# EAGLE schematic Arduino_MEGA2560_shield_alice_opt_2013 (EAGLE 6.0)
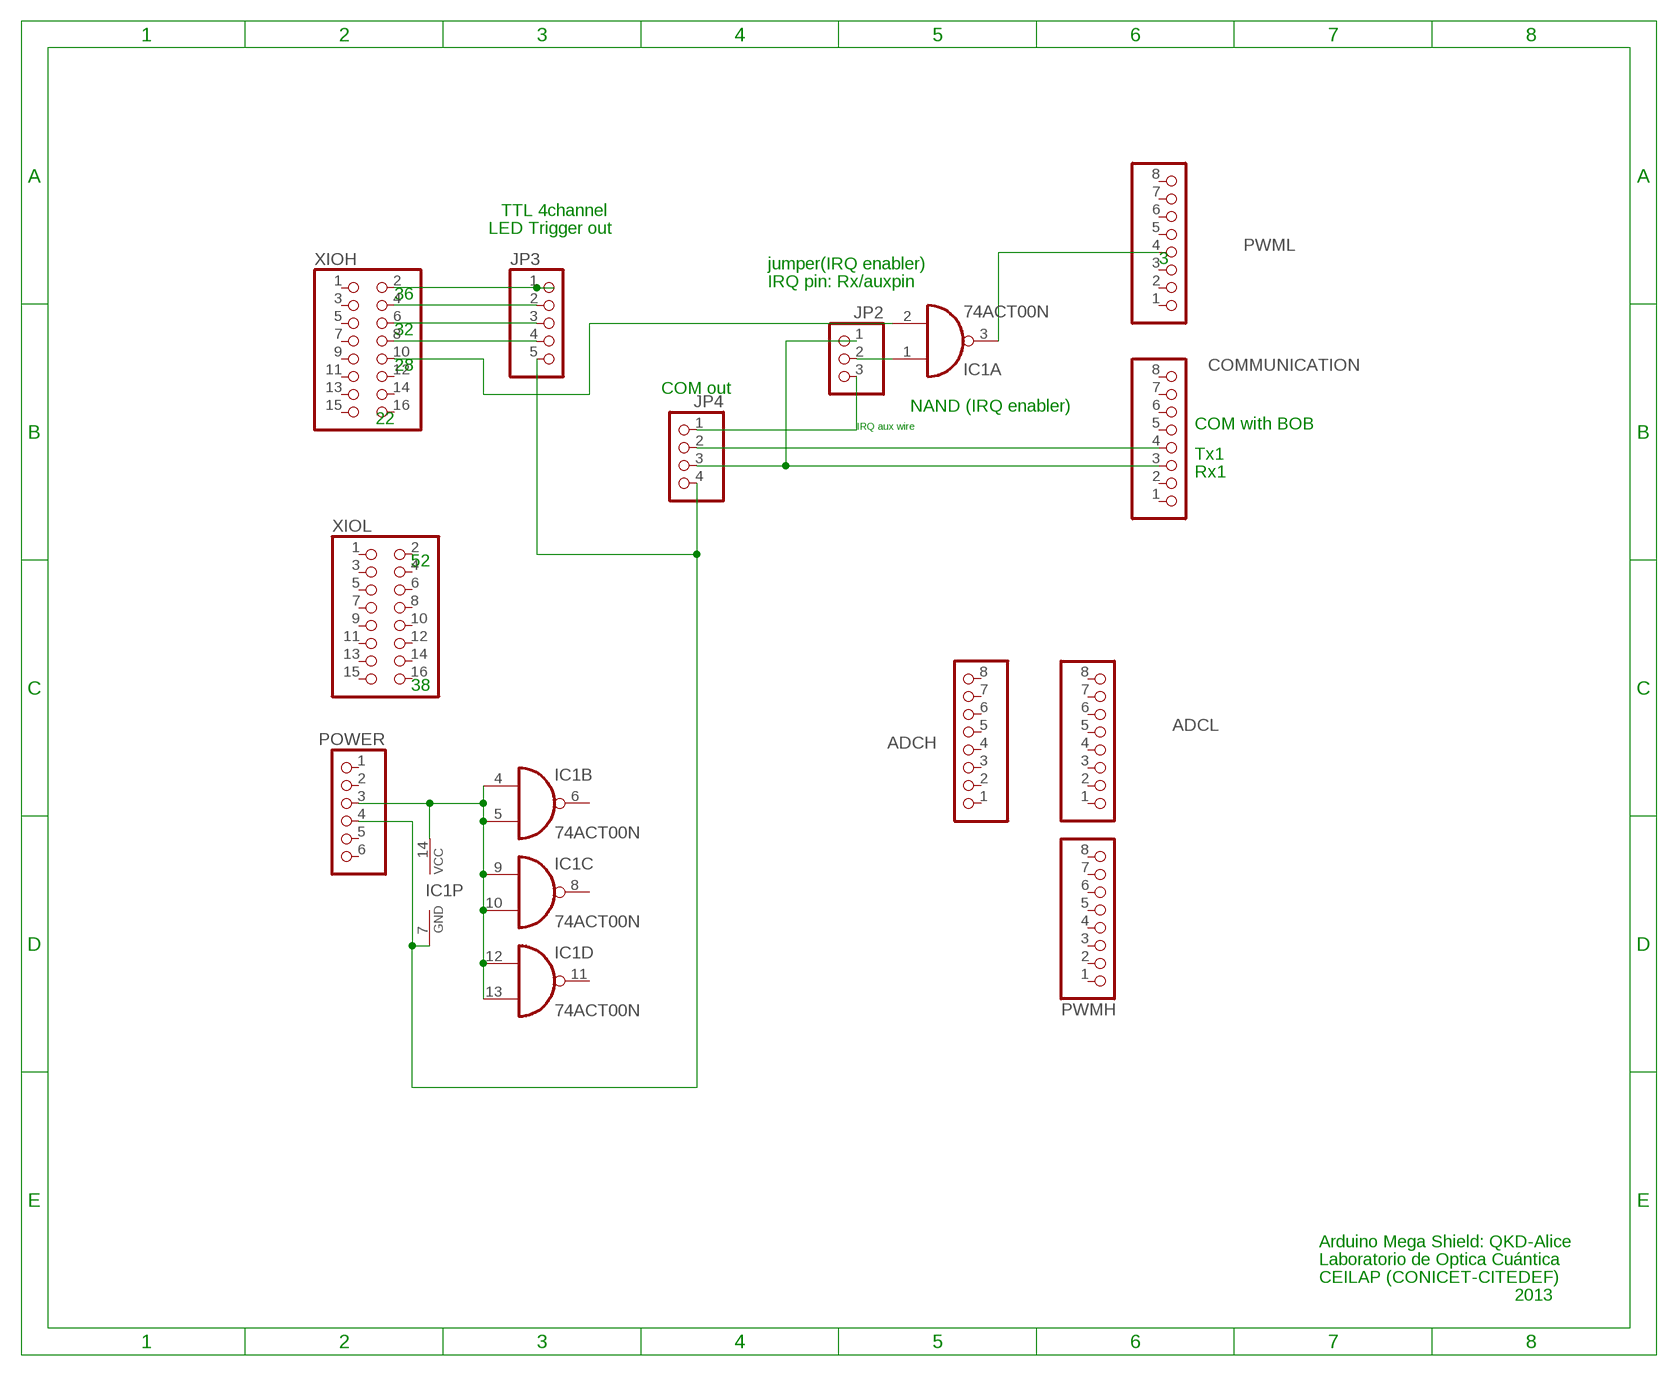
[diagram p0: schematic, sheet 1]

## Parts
ADCH  PINHD-1X8  [1X08]
ADCL  PINHD-1X8  [1X08]
COMMUNICATION  PINHD-1X8  [1X08]
IC1  74ACT00N  [DIL14]
JP2  PINHD-1X3  [1X03]
JP3  PINHD-1X5  [1X05]
JP4  PINHD-1X4  [1X04]
POWER  PINHD-1X6  [1X06]
PWMH  PINHD-1X8  [1X08]
PWML  PINHD-1X8  [1X08]
XIOH  PINHD-2X8  [2X08]
XIOL  PINHD-2X8  [2X08]

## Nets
GND: IC1.7(P:GND) JP3.5 JP4.4 POWER.4
N$1: IC1.1(A:I0) JP2.2
N$2: JP3.2 XIOH.4
N$3: JP3.3 XIOH.6
N$4: JP3.4 XIOH.8
N$5: IC1.2(A:I1) XIOH.10
N$6: JP3.1 XIOH.2
N$7: JP2.3 JP4.1
N$9: COMMUNICATION.4 JP4.2
N$10: COMMUNICATION.3 JP2.1 JP4.3
N$11: IC1.3(A:O) PWML.4
VCC: IC1.4(B:I0) IC1.5(B:I1) IC1.9(C:I0) IC1.10(C:I1) IC1.12(D:I0) IC1.13(D:I1) IC1.14(P:VCC) POWER.3
Unconnected: ADCH.1 ADCH.2 ADCH.3 ADCH.4 ADCH.5 ADCH.6 ADCH.7 ADCH.8 ADCL.1 ADCL.2 ADCL.3 ADCL.4 ADCL.5 ADCL.6 ADCL.7 ADCL.8 COMMUNICATION.1 COMMUNICATION.2 COMMUNICATION.5 COMMUNICATION.6 COMMUNICATION.7 COMMUNICATION.8 IC1.6(B:O) IC1.8(C:O) IC1.11(D:O) POWER.1 POWER.2 POWER.5 POWER.6 PWMH.1 PWMH.2 PWMH.3 PWMH.4 PWMH.5 PWMH.6 PWMH.7 PWMH.8 PWML.1 PWML.2 PWML.3 PWML.5 PWML.6 PWML.7 PWML.8 XIOH.1 XIOH.3 XIOH.5 XIOH.7 XIOH.9 XIOH.11 XIOH.12 XIOH.13 XIOH.14 XIOH.15 XIOH.16 XIOL.1 XIOL.2 XIOL.3 XIOL.4 XIOL.5 XIOL.6 XIOL.7 XIOL.8 XIOL.9 XIOL.10 XIOL.11 XIOL.12 XIOL.13 XIOL.14 XIOL.15 XIOL.16

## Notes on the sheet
- TTL 4channel
- LED Trigger out
- 3
- jumper(IRQ enabler)
- 36 | IRQ pin: Rx/auxpin
- 32
- 28
- COM out
- 22 | NAND (IRQ enabler)
- IRQ aux wire | COM with BOB
- Tx1
- Rx1
- 52
- 38
- Arduino Mega Shield: QKD-Alice
- Laboratorio de Optica Cuántica
- CEILAP (CONICET-CITEDEF)
- 2013

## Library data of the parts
ADCH ADCL COMMUNICATION PWMH PWML = pinhead:PINHD-1X8: PIN HEADER
IC1 = 74xx-eu:74*00: Quad 2-input NAND gate
JP2 = pinhead:PINHD-1X3: PIN HEADER
JP3 = pinhead:PINHD-1X5: PIN HEADER
JP4 = pinhead:PINHD-1X4: PIN HEADER
POWER = pinhead:PINHD-1X6: PIN HEADER
XIOH XIOL = pinhead:PINHD-2X8: PIN HEADER

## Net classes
0 default: width 0.152 mm, drill 0.305 mm, clearance 0.152 mm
